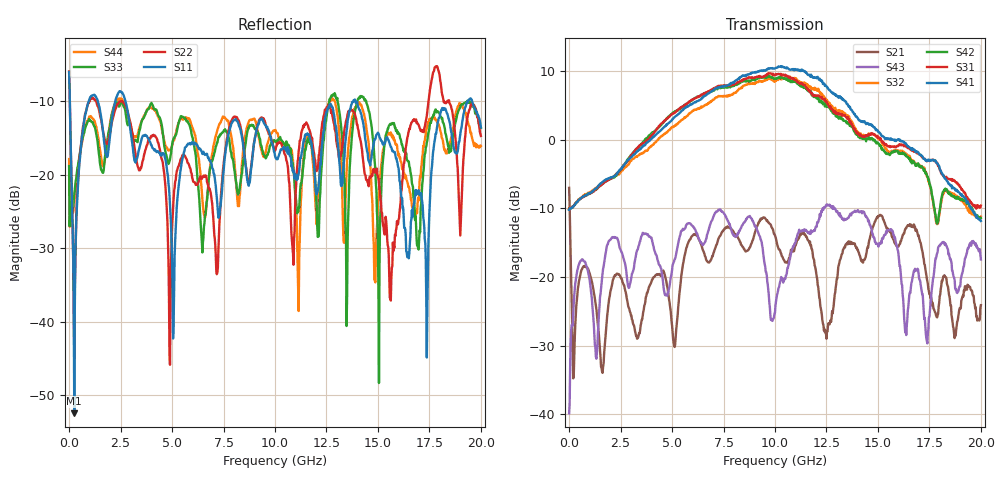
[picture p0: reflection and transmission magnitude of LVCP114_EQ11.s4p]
!Agilent Technologies,N5230A,MY46400459,A.07.50.48
!Agilent N5230A: A.07.50.48
!Date: Monday, January 09, 2012 14:03:25
!Correction: S11(Full 4 Port(1,2,3,4))
!S12(Full 4 Port(1,2,3,4))
!S13(Full 4 Port(1,2,3,4))
!S14(Full 4 Port(1,2,3,4))
!S21(Full 4 Port(1,2,3,4))
!S22(Full 4 Port(1,2,3,4))
!S23(Full 4 Port(1,2,3,4))
!S24(Full 4 Port(1,2,3,4))
!S31(Full 4 Port(1,2,3,4))
!S32(Full 4 Port(1,2,3,4))
!S33(Full 4 Port(1,2,3,4))
!S34(Full 4 Port(1,2,3,4))
!S41(Full 4 Port(1,2,3,4))
!S42(Full 4 Port(1,2,3,4))
!S43(Full 4 Port(1,2,3,4))
!S44(Full 4 Port(1,2,3,4))
!S4P File: Measurements: <S11,S12,S13,S14>,
!<S21,S22,S23,S24>,
!<S31,S32,S33,S34>,
!<S41,S42,S43,S44>:
# Hz S  dB  R 50
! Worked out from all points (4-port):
!   801 points, 300 kHz to 20 GHz, reference 50 ohm
!   strongest paths, dB at 300 kHz, 5 GHz, 10 GHz, 15 GHz, 20 GHz:
!     S41: -10.2, 2.9, 10.4, 1.3, -11.8
!     S31: -10.1, 3.7, 9.4, 0.3, -9.6
!     S42: -10.1, 3.8, 8.8, -0.5, -11.4
!     S32: -9.9, 1.8, 8.5, 0.2, -11.2
!     S43: -39.9, -19.0, -25.2, -15.2, -17.4
!     S21: -7.0, -27.1, -14.0, -11.1, -24.1
!   lowest |S11| = -52.4 dB at 250.3 MHz (marker M1), VSWR 1.00, Z = 50.2 - j0.052 ohm
!   |S11| at or under -10 dB: 34.38 MHz to 948.4 MHz (914 MHz wide, 186 % of centre); 2.738 GHz to 13.8 GHz (11.07 GHz wide, 134 % of centre); 13.91 GHz to 19.35 GHz (5.442 GHz wide, 32.7 % of centre)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
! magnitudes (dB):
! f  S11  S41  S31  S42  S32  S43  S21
! 300 kHz  -6.0  -10.2  -10.1  -10.1  -9.9  -39.9  -7.0
! 250.3 MHz  -52.4  -9.5  -9.6  -9.5  -9.5  -22.6  -31.3
! 1.15 GHz  -9.2  -7.5  -7.6  -7.5  -7.3  -24.9  -21.4
! 4.9 GHz  -24.1  2.6  3.5  3.5  1.5  -20.9  -24.2
! 8.025 GHz  -12.5  8.5  8.1  8.0  6.8  -14.0  -13.7
! 17.35 GHz  -37.5  -3.0  -3.0  -4.9  -4.9  -28.9  -19.7
! 20 GHz  -13.5  -11.8  -9.6  -11.4  -11.2  -17.4  -24.1
